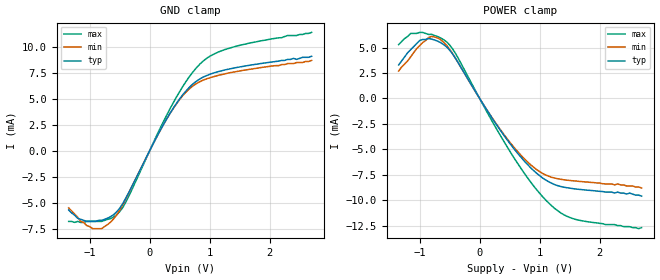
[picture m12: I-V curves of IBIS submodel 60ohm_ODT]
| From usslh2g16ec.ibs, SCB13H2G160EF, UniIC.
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| SUBMODEL 60ohm_ODT
[Submodel]   60ohm_ODT
Submodel_type  Dynamic_clamp
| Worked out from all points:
|   GND clamp passes 1 mA (typ) near -0.09 V on its own axis
|   POWER clamp passes 1 mA (typ) near -0.10 V on its own axis
[GND Clamp]
|Voltage   I(typ)   I(min)   I(max)
-1.35V    -5.7mA     -5.5mA     -6.8mA
-1.2V     -6.5mA     -6.4mA     -6.8mA
-950mV    -6.8mA     -7.5mA     -6.8mA
-800mV    -6.7mA     -7.5mA     -6.8mA
-650mV    -6.34mA    -6.86mA    -6.53mA
-400mV    -4.59mA    -4.65mA    -4.97mA
100mV     1.138mA    1.137mA    1.256mA
400mV     4.16mA     4.12mA     4.69mA
650mV     6.04mA     5.9mA      7.04mA
950mV     7.24mA     6.93mA     8.9mA
1.45V     8.02mA     7.63mA     10.08mA
2.7V      9.1mA      8.7mA      11.4mA
[POWER Clamp]
|Voltage   I(typ)   I(min)   I(max)
-1.35V    3.3mA      2.7mA      5.3mA
-1.15V    4.8mA      4.1mA      6.4mA
-1V       5.7mA      5.2mA      6.5mA
-850mV    5.9mA      6mA        6.3mA
-700mV    5.64mA     5.95mA     6.09mA
-550mV    5.07mA     5.22mA     5.56mA
-400mV    3.92mA     3.93mA     4.41mA
500mV     -4.4mA     -4.28mA    -5.15mA
850mV     -6.81mA    -6.52mA    -8.21mA
1.2V      -8.33mA    -7.75mA    -10.55mA
1.6V      -8.9mA     -8.11mA    -11.89mA
2.7V      -9.6mA     -8.8mA     -12.7mA
